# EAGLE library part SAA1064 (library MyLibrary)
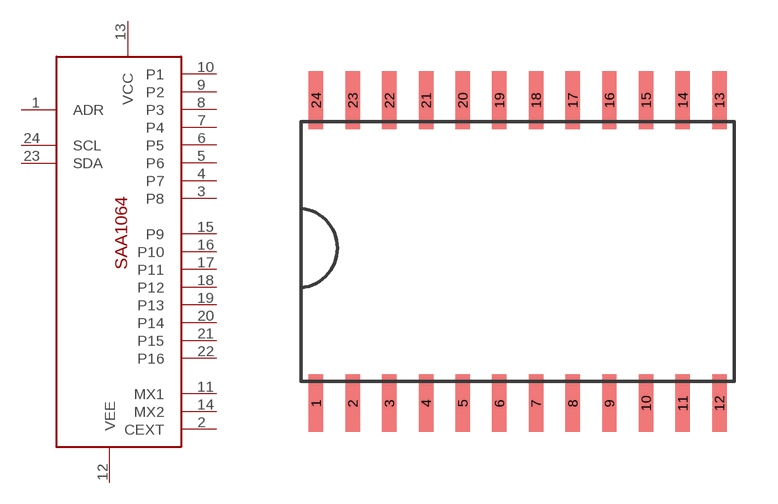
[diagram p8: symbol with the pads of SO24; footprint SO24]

Designator prefix -

## SAA1064  [SO24]
1  ADR
2  CEXT
3  P8
4  P7
5  P6
6  P5
7  P4
8  P3
9  P2
10  P1
11  MX1
12  VEE
13  VCC
14  MX2
15  P9
16  P10
17  P11
18  P12
19  P13
20  P14
21  P15
22  P16
23  SDA
24  SCL

## Footprint SO24 (pad centres in mm)
smd 0.5 x 2: 1 -6.985,-5.25; 2 -5.715,-5.25; 3 -4.445,-5.25; 4 -3.175,-5.25; 5 -1.905,-5.25; 6 -0.635,-5.25; 7 0.635,-5.25; 8 1.905,-5.25; 9 3.175,-5.25; 10 4.445,-5.25; 11 5.715,-5.25; 12 6.985,-5.25; 13 6.985,5.25; 14 5.715,5.25; 15 4.445,5.25; 16 3.175,5.25; 17 1.905,5.25; 18 0.635,5.25; 19 -0.635,5.25; 20 -1.905,5.25; 21 -3.175,5.25; 22 -4.445,5.25; 23 -5.715,5.25; 24 -6.985,5.25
